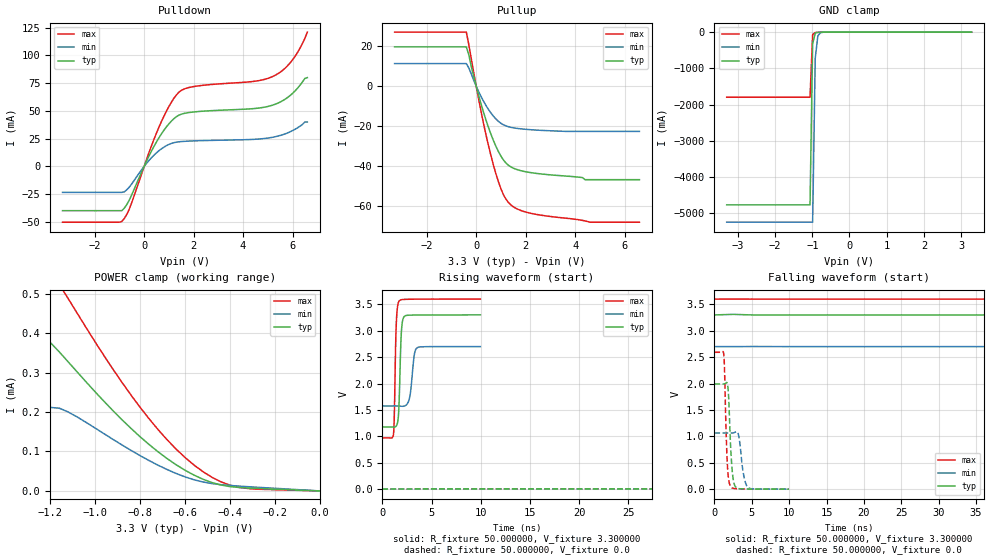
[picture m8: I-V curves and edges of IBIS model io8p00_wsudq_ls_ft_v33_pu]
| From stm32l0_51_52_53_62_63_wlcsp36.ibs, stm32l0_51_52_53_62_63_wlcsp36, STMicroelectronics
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|   Model io8p00_wsudq_ls_ft_v33_pu
[Model]  io8p00_wsudq_ls_ft_v33_pu
Model_type I/O
Polarity   Non-Inverting
Enable   Active-Low
Vinl =   0.990000V
Vinh =   2.310000V
Vmeas =  1.650000V
Cref =   50.000000pF
Rref =   100.000000M
Vref =   0.0V
C_comp   2.653200pF   2.620200pF   2.695100pF
[Temperature Range]   25.000000   0.125000k   -40.000000
[Pullup Reference]   3.300000V   2.700000V   3.600000V
[Pulldown Reference]   0.0V   0.0V   0.0V
[POWER Clamp Reference]   3.300000V   2.700000V   3.600000V
[GND Clamp Reference]   0.0V   0.0V   0.0V
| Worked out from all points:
|   slope of the pulldown table from 0 to 0.495 V, typ, clamps not added: 22.6 ohm
|   slope of the pullup table from 0 to 0.495 V, typ, clamps not added: 23.9 ohm
|   GND clamp passes 1 mA (typ) near -0.64 V on its own axis
|   POWER clamp passes 1 mA (typ) near -2.97 V on its own axis
|   rising waveform, R_fixture 50.000000, V_fixture 3.300000: 20-80 % time 213ps typ, 363ps min, 177ps max; typ from 1.18 V to 3.3 V
|   rising waveform, R_fixture 50.000000, V_fixture 0.0: 20-80 % time 204ns typ, 428ns min, 99.3ns max; typ from 0.001 V to 1.99 V
|   falling waveform, R_fixture 50.000000, V_fixture 3.300000: 20-80 % time 191ns typ, 378ns min, 105ns max; typ from 3.3 V to 1.18 V
|   falling waveform, R_fixture 50.000000, V_fixture 0.0: 20-80 % time 402ps typ, 571ps min, 325ps max; typ from 1.99 V to 0.001 V
[Pulldown]
|Voltage   I(typ)   I(min)   I(max)
-3.3V     -39.83mA   -23.36mA   -50.2mA
-900mV    -39.83mA   -23.36mA   -49.52mA
-600mV    -30.28mA   -18.58mA   -38.45mA
500mV     22.11mA    12.27mA    30.09mA
1V        38.33mA    19.81mA    53.88mA
1.4V      46.1mA     22.17mA    66.71mA
2V        49.06mA    23.01mA    71.93mA
4.4V      52.05mA    24.37mA    76.53mA
5.2V      55.25mA    26.3mA     81.02mA
6V        65.78mA    32.23mA    95.96mA
6.3V      73.07mA    36.19mA    106.4mA
6.6V      80mA       40mA       121mA
[Pullup]
|Voltage   I(typ)   I(min)   I(max)
-3.3V     19.79mA    11.39mA    27.22mA
-400mV    19.79mA    11.39mA    27.22mA
-300mV    15.85mA    9.195mA    20.96mA
-100mV    4.891mA    2.923mA    6.86mA
200mV     -9.111mA   -5.288mA   -12.97mA
600mV     -24.27mA   -13.54mA   -35.11mA
1V        -35.17mA   -18.65mA   -51.61mA
1.2V      -38.59mA   -19.95mA   -56.76mA
1.4V      -40.56mA   -20.67mA   -59.68mA
2.2V      -43.44mA   -21.87mA   -63.88mA
4.6V      -47mA      -22.71mA   -68.38mA
6.6V      -47mA      -22.71mA   -68.38mA
[GND_clamp]
|Voltage   I(typ)   I(min)   I(max)
-3.3V     -4.766A    -5.244A    -1.797A
-1.06V    -4.766A    -5.244A    -1.797A
-990mV    -326.7mA   -5.244A    -68.05mA
-920mV    -29.09mA   -722.2mA   -11.16mA
-850mV    -6.797mA   -104.4mA   -6.682mA
-780mV    -3.554mA   -17.44mA   -4.265mA
-500mV    -58.08uA   -169.3uA   -34.1uA
3.28V     0A         0A         0A
[POWER_clamp]
|Voltage   I(typ)   I(min)   I(max)
-3.28V    3.05A      226.6uA    3.724A
-2.96V    694.9uA    211.8uA    3.724A
-2.92V    479.6uA    211.8uA    509.1mA
-2.88V    432uA      211.8uA    70.08mA
-2.76V    412.8uA    211.8uA    794.1uA
-1.32V    411.6uA    211.8uA    593.3uA
-1.24V    395.5uA    211.8uA    578.2uA
-1.12V    327.2uA    200.2uA    487.6uA
-800mV    137.6uA    89.62uA    212.3uA
-560mV    40.27uA    28.42uA    65.81uA
-360mV    8.799uA    12.27uA    9.112uA
0V        0A         0A         0A
[Ramp]
| variable   typ   min   max
dV/dt_r  1.19492/0.20385u   0.61301/0.42830u   1.55547/99.10894n
dV/dt_f  1.27224/0.19119u   0.63594/0.37855u   1.57815/0.10498u
R_load = 50.000000
[Rising Waveform]
R_fixture= 50.000000
V_fixture= 3.300000
V_fixture_min= 2.700000
V_fixture_max= 3.600000
|time   V(typ)   V(min)   V(max)
0s        1.178V     1.575V     969.7mV
1.141ns   1.174V     1.576V     1.059V
1.221ns   1.174V     1.576V     1.442V
1.421ns   1.198V     1.575V     3.154V
1.702ns   1.645V     1.573V     3.561V
1.922ns   2.935V     1.57V      3.587V
2.222ns   3.269V     1.573V     3.593V
2.783ns   3.295V     1.744V     3.597V
3.483ns   3.297V     2.669V     3.598V
9.97ns    3.3V       2.7V       3.6V
[Rising Waveform]
R_fixture= 50.000000
V_fixture= 0.0
V_fixture_min= 0.0
V_fixture_max= 0.0
|time   V(typ)   V(min)   V(max)
0s        1.061mV    1.817mV    656.1uV
47.55ns   3.666mV    4.544mV    74.6mV
100.1ns   85.11mV    4.713mV    938.5mV
162.7ns   454.5mV    6.706mV    1.921V
202.7ns   744.2mV    21.57mV    2.286V
250.2ns   1.071V     56.75mV    2.478V
377.9ns   1.657V     231.8mV    2.579V
505.5ns   1.886V     455.3mV    2.591V
840.8ns   1.987V     894mV      2.593V
1.246us   1.993V     1.064V     2.593V
[Falling Waveform]
R_fixture= 50.000000
V_fixture= 3.300000
V_fixture_min= 2.700000
V_fixture_max= 3.600000
|time   V(typ)   V(min)   V(max)
0s        3.3V       2.7V       3.6V
85.09ns   3.3V       2.7V       3.461V
147.6ns   3.196V     2.7V       2.517V
207.7ns   2.865V     2.697V     1.629V
242.7ns   2.624V     2.688V     1.268V
277.8ns   2.373V     2.67V      1.099V
390.4ns   1.635V     2.55V      998.5mV
488ns     1.343V     2.389V     980.5mV
818.3ns   1.197V     1.799V     970.4mV
1.246us   1.178V     1.575V     969.7mV
[Falling Waveform]
R_fixture= 50.000000
V_fixture= 0.0
V_fixture_min= 0.0
V_fixture_max= 0.0
|time   V(typ)   V(min)   V(max)
0s        1.993V     1.064V     2.593V
1.241ns   1.992V     1.064V     2.562V
1.341ns   1.993V     1.064V     2.3V
1.722ns   2.001V     1.064V     489mV
1.902ns   1.733V     1.064V     182.9mV
2.142ns   875.4mV    1.064V     55.38mV
2.482ns   214.8mV    1.065V     17.75mV
2.923ns   30.56mV    1.09V      9.305mV
4.505ns   4.118mV    30.82mV    2.282mV
9.97ns    1.061mV    1.817mV    656.1uV
